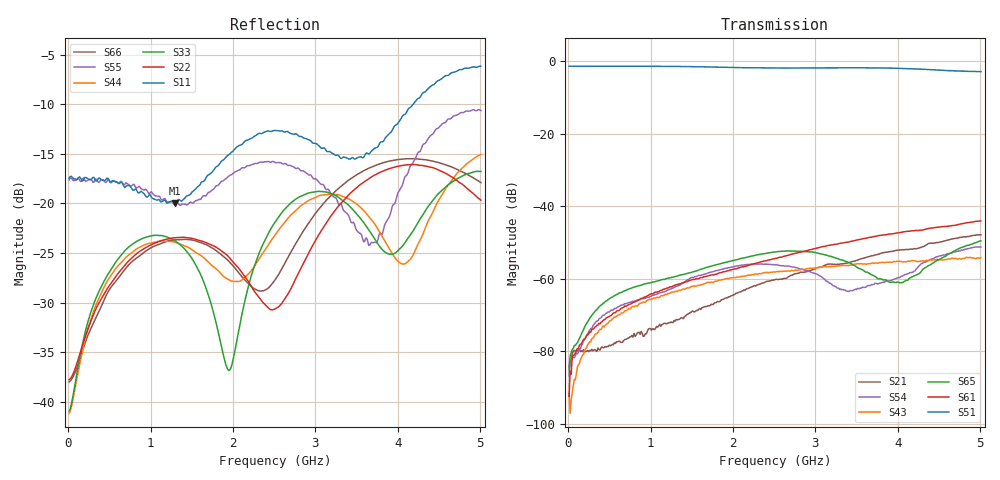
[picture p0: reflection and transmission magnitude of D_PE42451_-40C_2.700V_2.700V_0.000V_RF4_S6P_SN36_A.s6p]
! Device ID: PE42451
! Serial: 36
! Insertion: A
! Temp: -40C
! VDD: 2.700
! Control_Hi: 100.000
! Control_Lo: 0.000
! Logic State: RF4
! Port 1: RFC
! Port 2: RF1
! Port 3: RF2
! Port 4: RF3
! Port 5: RF4
! Port 6: RF5
! V1 = 0.00
! V2 = 0.00
! V3 = 2.70
! V4 = 0.00
! IDD: 1.078240e-05
#  Hz  S  RI  R  50
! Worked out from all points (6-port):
!   401 points, 10 MHz to 5.01 GHz, reference 50 ohm
!   strongest paths, dB at 10 MHz, 1.26 GHz, 2.51 GHz, 3.76 GHz, 5.01 GHz:
!     S51: -1.4, -1.4, -1.9, -1.9, -2.9
!     S61: -92.4, -62.2, -54.4, -48.1, -44.0
!     S65: -85.0, -59.5, -52.6, -60.0, -49.5
!     S43: -91.7, -63.6, -58.1, -55.7, -54.1
!     S54: -86.8, -62.6, -56.1, -61.4, -51.2
!     S21: -84.5, -72.0, -60.2, -53.2, -47.9
!   lowest |S11| = -20.0 dB at 1.298 GHz (marker M1), VSWR 1.22, Z = 53.6 - j9.81 ohm
!   |S11| at or under -10 dB: start of sweep to 4.187 GHz
